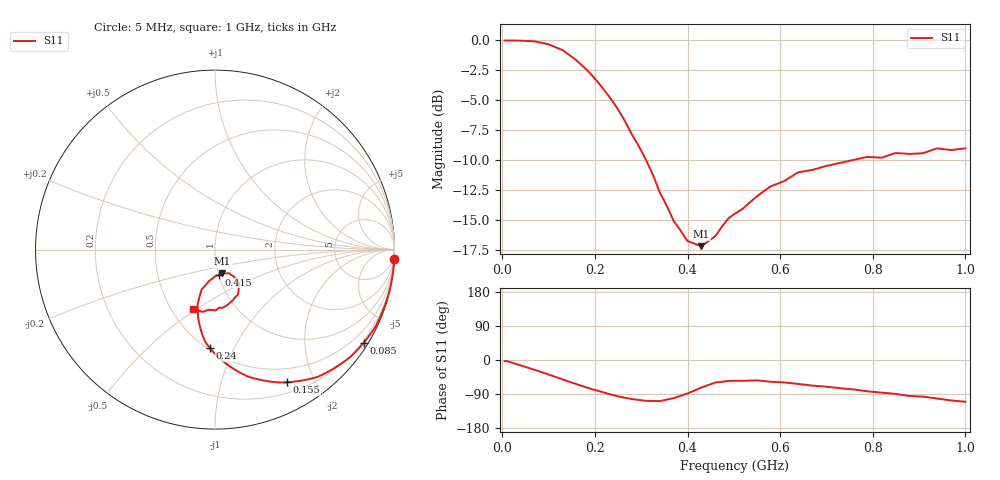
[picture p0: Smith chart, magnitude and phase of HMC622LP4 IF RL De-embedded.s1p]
! Hittite Microwave Corporation
! 20 Alpha Road
! Chelmsford, MA 01824
! http://www.hittite.com
! Tel: 978-250-3343
! Fax: 978-250-3373
! Device:  HMC622LP4
! Description:  GaAS MMIC MIXER With integrated IF/LO Amplifier
! Frequency:  1.8-  3.9 GHz
! Package:
! Data:  The device was measured on evaluation board 119242
!  The evaluation circuit board was modeled and simulated.  This was use
!  to removed the evaluation board circuit from the measured data.
!  The reference plane is the center of the package pin.
! Misc:
! Date Measured:  06-09-2009
! Date:  08-24-2009
! Note:
!  Hittite supplies this data as a sample of measured data at the package pin for
!  for this package product.  Your particular data for this product may vary.
!  Data was taken at 25 degrees C.
!  Hittite reserves the right to change this data at anytime
# MHz S MA R 50
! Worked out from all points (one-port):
!   200 points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, 5 MHz to 1 GHz, reference 50 ohm
!   lowest |S11| = -17.2 dB at 430 MHz (marker M1), VSWR 1.32, Z = 52.4 - j14.1 ohm
!   |S11| at or under -10 dB: 310.7 MHz to 755.7 MHz (445 MHz wide, 83.5 % of centre)
!   S11 on the Smith chart (normalised r, x): 5 MHz: -0, -37; 85 MHz: 0.15, -3.48; 155 MHz: 0.32, -1.63; 240 MHz: 0.51, -0.81; 415 MHz: 1.01, -0.29; 1 GHz: 0.64, -0.49
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5  1 -3.1
10  1 -3.0
45  0.9976 -16.3
70  0.9916 -25.9
85  0.9777 -32.0
105  0.9549 -40.3
130  0.9112 -51.1
155  0.8408 -61.6
190  0.729 -75.6
215  0.639 -84.4
240  0.5507 -92.8
255  0.4969 -97.3
280  0.4044 -103.1
310  0.3182 -107.7
340  0.2325 -108.5
380  0.1661 -96.5
400  0.1454 -88.3
415  0.1418 -80.4
430  0.1385 -72.6
460  0.1524 -59.4
490  0.1823 -55.1
505  0.1905 -55.0
550  0.2236 -53.7
630  0.2749 -61.9
755  0.316 -77.2
880  0.3361 -95.1
940  0.3543 -102.0
1000  0.3544 -110.2
